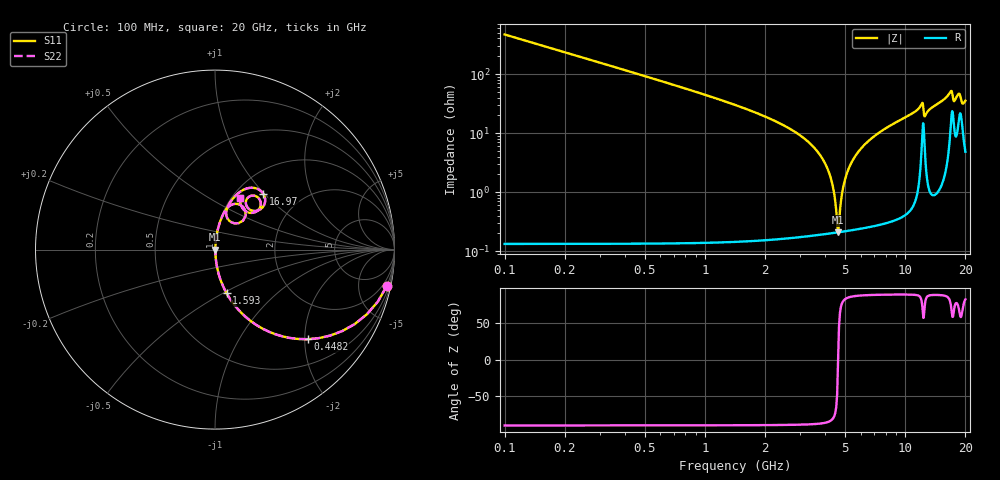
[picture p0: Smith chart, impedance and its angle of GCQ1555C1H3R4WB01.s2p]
!Murata Part Number: GCQ1555C1H3R4WB01
!These Parameters are Measured in Series Mode Connection
!Data Generated on Jan 08, 2026
!  o--ll--o
!Port1  Port2
!  o------o
!Operation Temp=25[degC], DC Bias Voltage=0[V]
!Freq. Start=100[MHz] Stop=20[GHz] 401[Steps]
# Hz S RI R 50
!Freq.(Hz) S11(Real) S11(Imag) S21(Real) S21(Imag) S12(Real) S12(Imag) S22(Real) S22(Imag)
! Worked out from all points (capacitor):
!   401 points, 100 MHz to 20 GHz, reference 50 ohm
!   read as one part in series: C = 3.4 pF near 199.5 MHz
!   lowest |Z| = 209 mohm at 4.627 GHz (marker M1)
!   series resonance near 4.628 GHz, so ESL is about 350 pH
!   S11 on the Smith chart (normalised r, x): 100 MHz: 1.00, -9.36; 448.2 MHz: 1.00, -2.07; 1.593 GHz: 1.00, -0.52; 16.97 GHz: 1.31, +0.99; 20 GHz: 1.10, +0.70
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1e8  0.9563 -0.2044  0.0437 0.2044  0.0437 0.2044  0.9563 -0.2044
4.4825e8  0.517 -0.4991  0.483 0.4991  0.483 0.4991  0.517 -0.4991
8.96e8  0.2025 -0.4005  0.7975 0.4005  0.7975 0.4005  0.2025 -0.4005
1.5925e9  0.0642 -0.2423  0.9358 0.2423  0.9358 0.2423  0.0642 -0.2423
3.43325e9  0.00558 -0.0611  0.9944 0.0611  0.9944 0.0611  0.00558 -0.0611
4.1795e9  0.00241 -0.0207  0.9976 0.0207  0.9976 0.0207  0.00241 -0.0207
4.3785e9  0.00216 -0.0113  0.9978 0.0113  0.9978 0.0113  0.00216 -0.0113
4.62725e9  0.00208 -4.76e-05  0.9979 4.76e-05  0.9979 4.76e-05  0.00208 -4.76e-05
4.92575e9  0.00231 0.0127  0.9977 -0.0127  0.9977 -0.0127  0.00231 0.0127
5.274e9  0.00294 0.0267  0.9971 -0.0267  0.9971 -0.0267  0.00294 0.0267
5.871e9  0.00477 0.049  0.9952 -0.049  0.9952 -0.049  0.00477 0.049
6.7665e9  0.00897 0.0795  0.991 -0.0795  0.991 -0.0795  0.00897 0.0795
1.005e10  0.0372 0.1785  0.9628 -0.1785  0.9628 -0.1785  0.0372 0.1785
1.208975e10  0.126 0.2541  0.874 -0.2541  0.874 -0.2541  0.126 0.2541
1.25375e10  0.0785 0.1618  0.9215 -0.1618  0.9215 -0.1618  0.0785 0.1618
1.338325e10  0.0706 0.2382  0.9294 -0.2382  0.9294 -0.2382  0.0706 0.2382
1.67165e10  0.2249 0.3422  0.7751 -0.3422  0.7751 -0.3422  0.2249 0.3422
1.696525e10  0.2685 0.3121  0.7315 -0.3121  0.7315 -0.3121  0.2685 0.3121
1.75125e10  0.1875 0.2275  0.8125 -0.2275  0.8125 -0.2275  0.1875 0.2275
1.845775e10  0.2376 0.2918  0.7624 -0.2918  0.7624 -0.2918  0.2376 0.2918
1.925375e10  0.1759 0.2107  0.8241 -0.2107  0.8241 -0.2107  0.1759 0.2107
2e10  0.142 0.2869  0.858 -0.2869  0.858 -0.2869  0.142 0.2869
